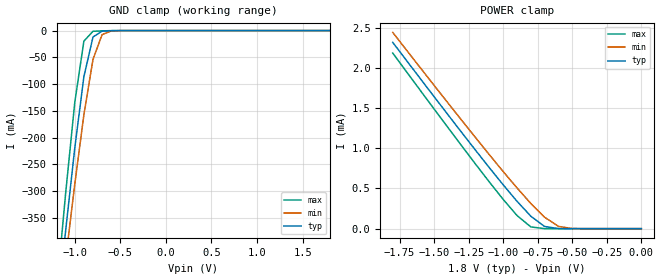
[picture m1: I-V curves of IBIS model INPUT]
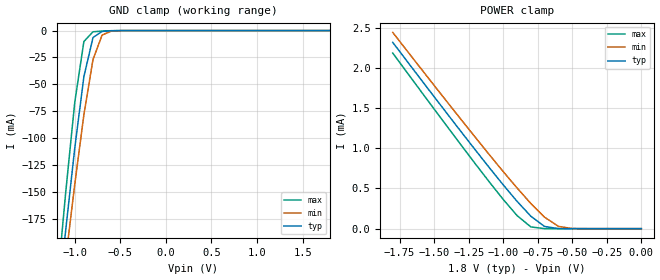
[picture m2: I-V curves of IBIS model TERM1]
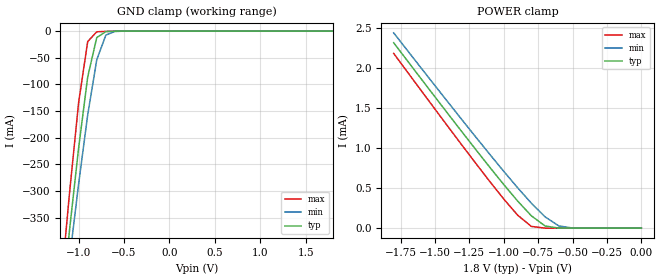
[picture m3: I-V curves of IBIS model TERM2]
|   PERICOM SEMICONDUCTOR CORP
|   IBIS Model of PI4MSD5V9546A
|   Product Family: 4MSD
|   SOIC-16 (W) Package
[IBIS Ver] 3.2
[Comment char] |_char
[File Name] pi4msd5v9546a_w_18v.ibs
[File Rev] 1.0
[Source] File originated at Pericom Semiconductor Corp.
[Date] 09/07/17
[Disclaimer] (C) Copyright PERICOM Semiconductor Corporation
   All rights reserved
  Pericom Semiconductor Corporation hereby grants the user of
  this IBIS model a non-exclusive, nontransferable license to
  use this IBIS model under the following terms.
  This IBIS model is provided on an "AS IS" basis and Pericom
  makes absolutely no warranty with respect to the information
  contained herein. PERICOM DISCLAIMS AND CUSTOMER WAIVES ALL
  WARRANTIES, EXPRESSED OR IMPLIED, INCLUDING WARRANTIES OF
  MERCHANTABILITY OR FITNESS FOR A PARTICULAR PURPOSE. The
  entire risk as to quality and performance is with the customer.
  Accordingly, in no event shall the company be liable for any
  damages, whether in contract or tort, including any lost
  profits or other incidental, consequential, exemplary, or
  punitive damages arising out of the use or application of the
  IBIS model provided in this package. Further, Pericom reserves
  the right to make changes without notice to any product herein
  to improve reliability, function, or design. Pericom does not
  convey any license under patent rights or any other intellectual
  property rights, including those of third parties.
  The user is granted this license only to use the IBIS model
  and is not granted rights to sell, load, rent, lease or license
  the IBIS model in whole or in part, or in modified form to anyone
  other than user. User may modify the IBIS model to suit its specific
  application but rights to derivative works and such modifications
  shall belong to Pericom.
  Pericom is not obligated to provide maintenance or support
  for the licensed IBIS model.
  Contact Pericom at ATTN: APPLICATION ENGINEERING / IBIS MODELS
  2380 Bering Drive, San Jose, CA 95131
[Component] PI4MSD5V9546A
[Manufacturer] Pericom Semiconductor Corp.
[Package]
| variable   typ   min   max
R_pkg   0.05665ohm   0.05334ohm   0.05997ohm
L_pkg   1.99150nH   1.82200nH   2.76100nH
C_pkg   0.20800pF   0.16300pF   0.25300pF
[Pin] signal_name   model_name   R_pin   L_pin   C_pin
1   A0   INPUT   0.05997   2.76100nH   0.25300pF
2   A1   INPUT   0.05776   2.54800nH   0.22300pF
3   _RESET   INPUT   0.05555   2.33500nH   0.19300pF
4   SD0   TERM1   0.05334   2.12200nH   0.16300pF
5   SC0   TERM1   0.05334   2.12200nH   0.16300pF
6   SD1   TERM1   0.05555   2.33500nH   0.19300pF
7   SC1   TERM1   0.05776   2.54800nH   0.22300pF
8   GND   GND   0.05997   2.76100nH   0.25300pF
9   SD2   TERM1   0.05997   2.76100nH   0.25300pF
10   SC2   TERM1   0.05776   2.54800nH   0.22300pF
11   SD3   TERM1   0.05555   2.33500nH   0.19300pF
12   SC3   TERM1   0.05334   2.12200nH   0.16300pF
13   A2   INPUT   0.05334   2.12200nH   0.16300pF
14   SCL   TERM2   0.05555   2.33500nH   0.19300pF
15   SDA   TERM2   0.05776   2.54800nH   0.22300pF
16   VCC   POWER   0.05997   2.76100nH   0.25300pF
[Series Switch Groups]
On 1 /
Off 2 3 4 /
[Series Pin Mapping]   pin_2   model_name  function_table_group
4   15   SWITCH1   1
5   14   SWITCH1   1
6   15   SWITCH1   2
7   14   SWITCH1   2
9   15   SWITCH1   3
10   14   SWITCH1   3
11   15   SWITCH1   4
12   14   SWITCH1   4
|   Model SWITCH1
[Model] SWITCH1
Model_type Series_switch
| variable   typ   min   max
C_comp   7.10pF   7.08pF   7.12pF
[Voltage Range]   1.8000V   1.6200V   1.9800V
[GND Clamp Reference]   0.0000V   0.0000V   0.0000V
[POWER Clamp Reference]   1.8000V   1.6200V   1.9800V
[Temperature Range]   25   85   -40
[On]
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[OFF]
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| Models and submodels in the file (4): INPUT (Input), SWITCH1 (Series_switch), TERM1 (Terminator), TERM2 (Terminator)
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|   Model INPUT
[Model] INPUT
Model_type Input
Vinl = 540mV
Vinh = 1.26V
| variable   typ   min   max
C_comp   4.45pF   4.44pF   4.46pF
[Voltage Range]   1.8000V   1.6200V   1.9800V
[GND Clamp Reference]   0.0000V   0.0000V   0.0000V
[POWER Clamp Reference]   1.8000V   1.6200V   1.9800V
[Temperature Range]   25   85   -40
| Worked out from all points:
|   GND clamp passes 1 mA (typ) near -0.70 V on its own axis
|   POWER clamp passes 1 mA (typ) near -1.21 V on its own axis
[GND Clamp]
| Voltage   I(typ)   I(min)   I(max)
-1.8V     -1.564A    -1.492A    -1.669A
-1.2V     -536.3mA   -573.9mA   -488.8mA
-1.1V     -373.8mA   -427.8mA   -304mA
-1V       -219.8mA   -287.2mA   -134.4mA
-900mV    -86.22mA   -157.4mA   -19.74mA
-800mV    -12.06mA   -53.77mA   -1.311mA
-700mV    -1.032mA   -7.522mA   -526.9uA
-600mV    -210.6uA   -734.5uA   -129.9uA
1.8V      68.64pA    148.9pA    67.17pA
[POWER Clamp]   |Note: Vtable = Vcc - Voutput
| Voltage   I(typ)   I(min)   I(max)
-1.8V     2.317mA    2.441mA    2.184mA
-1.4V     1.417mA    1.564mA    1.257mA
-1.1V     757.6uA    919.3uA    579.7uA
-1V       544.9uA    710.2uA    363.8uA
-900mV    340.5uA    506.6uA    163.7uA
-800mV    155.1uA    313.2uA    21.83uA
-700mV    27.01uA    141.6uA    235.7nA
-600mV    852.4nA    28.01uA    1.729nA
-500mV    17.68nA    1.596uA    108.9pA
0V        68.64pA    88.42pA    75.24pA
|   Model TERM1
[Model] TERM1
Model_type Terminator
| variable   typ   min   max
C_comp   2.65pF   2.64pF   2.66pF
[Voltage Range]   1.8000V   1.6200V   1.9800V
[GND Clamp Reference]   0.0000V   0.0000V   0.0000V
[POWER Clamp Reference]   1.8000V   1.6200V   1.9800V
[Temperature Range]   25   85   -40
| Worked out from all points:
|   GND clamp passes 1 mA (typ) near -0.70 V on its own axis
|   POWER clamp passes 1 mA (typ) near -1.21 V on its own axis
[GND Clamp]
| Voltage   I(typ)   I(min)   I(max)
-1.8V     -779.5mA   -743.6mA   -831.9mA
-1.2V     -267.2mA   -286mA     -243.4mA
-1.1V     -186.2mA   -213.2mA   -151.2mA
-1V       -109.4mA   -143.1mA   -66.79mA
-900mV    -42.98mA   -78.43mA   -10.22mA
-800mV    -6.45mA    -26.94mA   -1.105mA
-700mV    -805uA     -4.15mA    -477.3uA
-600mV    -185.9uA   -544.9uA   -115.7uA
1.8V      37.5pA     93.35pA    36.54pA
[POWER Clamp]   |Note: Vtable = Vcc - Voutput
| Voltage   I(typ)   I(min)   I(max)
-1.8V     2.317mA    2.441mA    2.184mA
-1.4V     1.417mA    1.564mA    1.257mA
-1.1V     757.6uA    919.3uA    579.7uA
-1V       544.9uA    710.2uA    363.8uA
-900mV    340.5uA    506.6uA    163.7uA
-800mV    155.1uA    313.2uA    21.83uA
-700mV    27.01uA    141.6uA    235.6nA
-600mV    852.4nA    28.01uA    1.684nA
-500mV    17.64nA    1.596uA    65.36pA
0V        37.5pA     37.78pA    41.21pA
|   Model TERM2
[Model] TERM2
Model_type Terminator
| variable   typ   min   max
C_comp   4.45pF   4.44pF   4.46pF
[Voltage Range]   1.8000V   1.6200V   1.9800V
[GND Clamp Reference]   0.0000V   0.0000V   0.0000V
[POWER Clamp Reference]   1.8000V   1.6200V   1.9800V
[Temperature Range]   25   85   -40
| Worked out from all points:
|   GND clamp passes 1 mA (typ) near -0.70 V on its own axis
|   POWER clamp passes 1 mA (typ) near -1.21 V on its own axis
[GND Clamp]
| Voltage   I(typ)   I(min)   I(max)
-1.8V     -1.564A    -1.492A    -1.669A
-1.2V     -536.3mA   -573.9mA   -488.8mA
-1.1V     -373.8mA   -427.8mA   -304mA
-1V       -219.8mA   -287.2mA   -134.4mA
-900mV    -86.22mA   -157.4mA   -19.74mA
-800mV    -12.06mA   -53.77mA   -1.311mA
-700mV    -1.032mA   -7.522mA   -526.9uA
-600mV    -210.6uA   -734.5uA   -129.9uA
1.8V      68.64pA    148.9pA    67.17pA
[POWER Clamp]   |Note: Vtable = Vcc - Voutput
| Voltage   I(typ)   I(min)   I(max)
-1.8V     2.317mA    2.441mA    2.184mA
-1.4V     1.417mA    1.564mA    1.257mA
-1.1V     757.6uA    919.3uA    579.7uA
-1V       544.9uA    710.2uA    363.8uA
-900mV    340.5uA    506.6uA    163.7uA
-800mV    155.1uA    313.2uA    21.83uA
-700mV    27.01uA    141.6uA    235.7nA
-600mV    852.4nA    28.01uA    1.729nA
-500mV    17.68nA    1.596uA    108.9pA
0V        68.64pA    88.42pA    75.24pA
